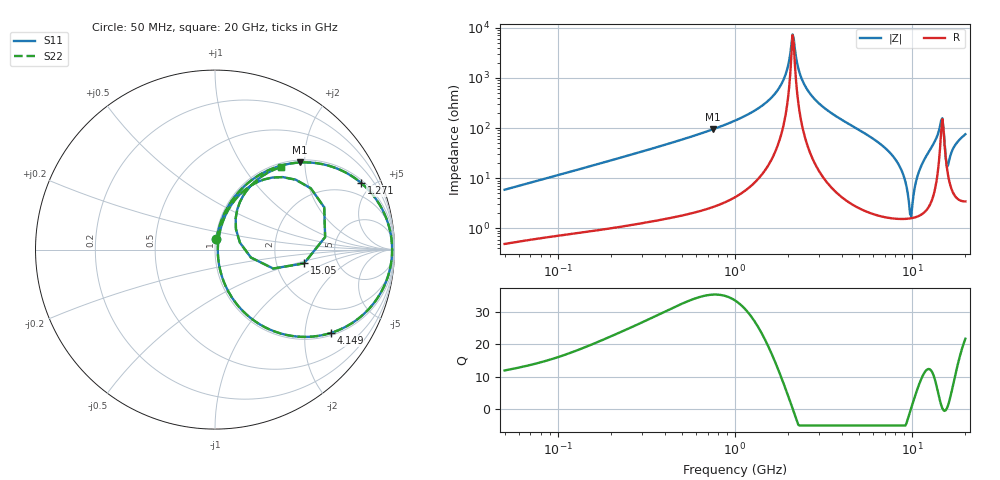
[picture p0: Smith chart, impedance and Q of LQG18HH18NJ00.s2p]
!Murata Part Number: LQG18HH18NJ00
!These Parameters are Measured in Series Mode Connection
!  o--[Z]--o
!Port1  Port2
!  o-------o
!Freq. Start=50[MHz] Stop=20[GHz], 401[Steps]
# Hz S RI R 50
!Freq.(Hz) S11(Real) S11(Imag) S21(Real) S21(Imag) S12(Real) S12(Imag) S22(Real) S22(Imag)
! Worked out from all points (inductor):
!   401 points, 50 MHz to 20 GHz, reference 50 ohm
!   read as one part in series: L = 18.5 nH near 51.52 MHz
!   highest Q = 35.4 at 752.3 MHz (marker M1), where L = 20 nH
!   self-resonance near 2.115 GHz
!   S11 on the Smith chart (normalised r, x): 50 MHz: 1.01, +0.12; 1.271 GHz: 1.16, +4.30; 4.149 GHz: 1.08, -2.71; 15.05 GHz: 2.88, -0.59; 20 GHz: 1.07, +1.50
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5e7  0.00828 0.058  0.9917 -0.058  0.9917 -0.058  0.00828 0.058
1.364002e8  0.0313 0.1496  0.9687 -0.1496  0.9687 -0.1496  0.0313 0.1496
3.721004e8  0.1629 0.3526  0.8371 -0.3526  0.8371 -0.3526  0.1629 0.3526
7.523192e8  0.4734 0.4854  0.5266 -0.4854  0.5266 -0.4854  0.4734 0.4854
1e9  0.6595 0.4592  0.3405 -0.4592  0.3405 -0.4592  0.6595 0.4592
1.270815e9  0.8136 0.3718  0.1864 -0.3718  0.1864 -0.3718  0.8136 0.3718
1.793498e9  0.9656 0.1422  0.0344 -0.1422  0.0344 -0.1422  0.9656 0.1422
1.932977e9  0.9802 0.0804  0.0198 -0.0804  0.0198 -0.0804  0.9802 0.0804
2.114743e9  0.9869 0.00333  0.0131 -0.00333  0.0131 -0.00333  0.9869 0.00333
2.383959e9  0.9764 -0.1011  0.0236 0.1011  0.0236 0.1011  0.9764 -0.1011
2.728004e9  0.9369 -0.2153  0.0631 0.2153  0.0631 0.2153  0.9369 -0.2153
4.149438e9  0.644 -0.4649  0.356 0.4649  0.356 0.4649  0.644 -0.4649
7.442007e9  0.1105 -0.2901  0.8895 0.2901  0.8895 0.2901  0.1105 -0.2901
8.774992e9  0.0323 -0.1288  0.9677 0.1288  0.9677 0.1288  0.0323 -0.1288
9.892087e9  0.0157 0.00687  0.9843 -0.00687  0.9843 -0.00687  0.0157 0.00687
1.066139e10  0.0264 0.0966  0.9736 -0.0966  0.9736 -0.0966  0.0264 0.0966
1.166392e10  0.0663 0.2076  0.9337 -0.2076  0.9337 -0.2076  0.0663 0.2076
1.396067e10  0.3773 0.4039  0.6227 -0.4039  0.6227 -0.4039  0.3773 0.4039
1.504638e10  0.4963 -0.0765  0.5037 0.0765  0.5037 0.0765  0.4963 -0.0765
1.597544e10  0.1166 0.1145  0.8834 -0.1145  0.8834 -0.1145  0.1166 0.1145
1.747767e10  0.193 0.3486  0.807 -0.3486  0.807 -0.3486  0.193 0.3486
2e10  0.3675 0.4597  0.6325 -0.4597  0.6325 -0.4597  0.3675 0.4597
